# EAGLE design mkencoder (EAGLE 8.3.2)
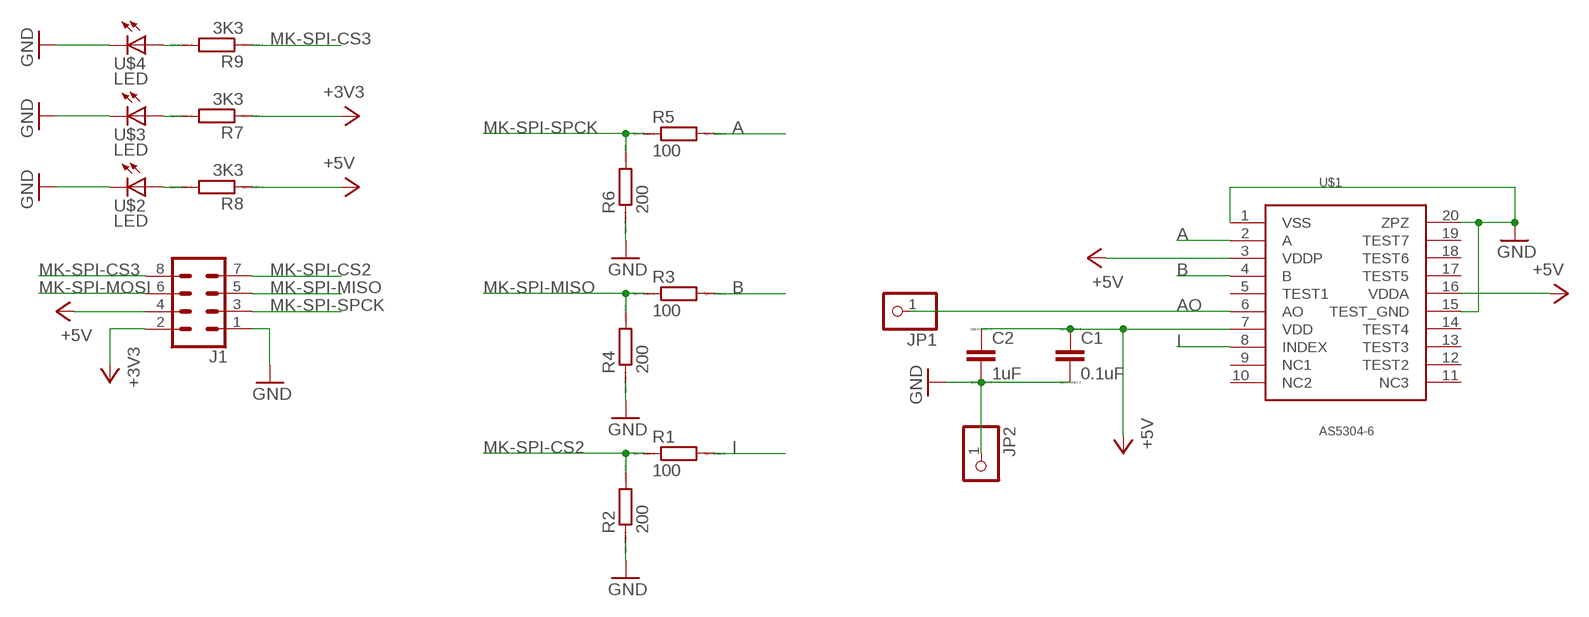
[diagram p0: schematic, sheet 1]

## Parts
C1  0.1uF  C  [C0805]
C2  1uF  C  [C0805]
J1  CONN_04X2SHROUDED-SQUISH  [2X4-SHROUDED-SQUISH]
JP1  PINHD-1X1  [1X01]
JP2  PINHD-1X1  [1X01]
R1  100  RR1206  [R1206]
R2  200  RR1206  [R1206]
R3  100  RR1206  [R1206]
R4  200  RR1206  [R1206]
R5  100  RR1206  [R1206]
R6  200  RR1206  [R1206]
R7  3K3  RR1206  [R1206]
R8  3K3  RR1206  [R1206]
R9  3K3  RR1206  [R1206]
U$1  AS5304-6  [TSSOP20-08THIN]
U$2  LED  [LED1206]
U$3  LED  [LED1206]
U$4  LED  [LED1206]

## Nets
+3V3: J1.2 R7.1
+5V: C1.1 C2.1 J1.4 R8.1 U$1.3(VDDP) U$1.7(VDD) U$1.16(VDDA)
A: R5.2 U$1.2(A)
AO: JP1.1 U$1.6(AO)
B: R3.2 U$1.4(B)
GND: C1.2 C2.2 J1.1 JP2.1 R2.1 R4.1 R6.1 U$1.1(VSS) U$1.15(TEST_GND) U$1.20(ZPZ) U$2.2(C) U$3.2(C) U$4.2(C)
I: R1.2 U$1.8(INDEX)
MK-SPI-CS2: J1.7 R1.1 R2.2
MK-SPI-CS3: J1.8 R9.1
MK-SPI-MISO: J1.5 R3.1 R4.2
MK-SPI-MOSI: J1.6
MK-SPI-SPCK: J1.3 R5.1 R6.2
N$1: R8.2 U$2.1(A)
N$2: R7.2 U$3.1(A)
N$5: R9.2 U$4.1(A)
Unconnected: U$1.5(TEST1) U$1.9(NC1) U$1.10(NC2) U$1.11(NC3) U$1.12(TEST2) U$1.13(TEST3) U$1.14(TEST4) U$1.17(TEST5) U$1.18(TEST6) U$1.19(TEST7)

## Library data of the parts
C1 C2 = eagle-ltspice:C: CAPACITOR, European symbol; SPICEMODEL: NONE; SPICEPREFIX: C
J1 = fab:CONN_04X2: Multi connection point. Often used as Generic Header-pin footprint for 0.1 inch spaced/style header connections On any of the 0.1 inch spaced packages, you can populate with these: Break Away Headers - Straight (PRT-00116) Break Away Male Headers - Right Angle (PRT-00553) Female Headers (PRT-00115)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
JP1 JP2 = pinhead:PINHD-1X1: PIN HEADER
R1-R9 = eagle-ltspice:R: RESISTOR, European symbol; SPICEMODEL: NONE; SPICEPREFIX: R
U$1 = fab:AS5304-6
U$2-U$4 = fab:LED: LED

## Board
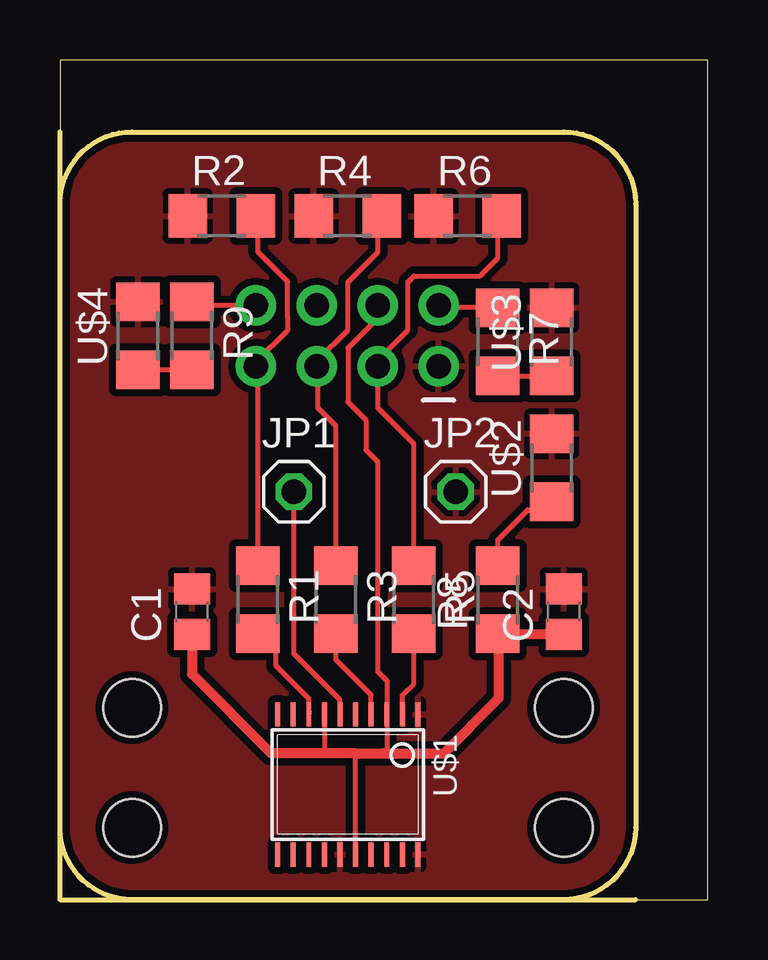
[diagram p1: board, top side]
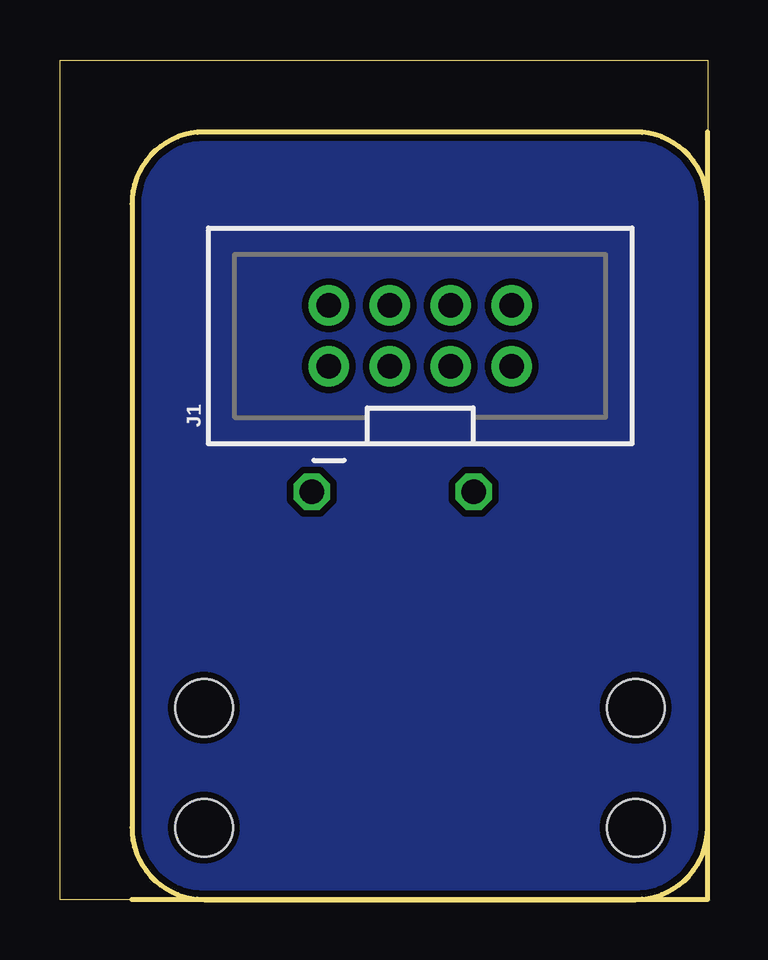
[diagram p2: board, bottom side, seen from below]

Size 27 x 35 mm. Coordinates in mm from the lower left corner, seen from the top.
Outline: 0,3 0,0 3,0
Outline: 0,3 0,29
Outline: 0,29 0,32 0,35 27,35 27,0 24,0 21,0
Outline: 3,0 21,0
Outline: 0,29 arc-90 3,32 21,32 arc-90 24,29 24,3 arc-90 21,0
Outline: 3,0 arc-90 0,3
Copper layers (1*16): Top 0.035mm / dielectric 1.5mm / Bottom 0.035mm
Design rules "default *": minimum track width 7mil, minimum drill 0.35mm, track to track 11mil, track to pad 11mil, pad to pad 11mil, via to via 11mil, smd to smd 11mil, copper to edge 11mil, drill to drill 11mil, minimum pad ring 10mil, minimum via ring 8mil, stop-mask expansion 4mil, vias tented up to drill 0mil, thermal gap 10mil
Holes 2.4 mm at 3,3 21,3 3,8 21,8
Milling: 8 lines

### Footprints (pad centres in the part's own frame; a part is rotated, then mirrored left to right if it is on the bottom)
C0805 = smd 1.3 x 1.5: 1 -0.95,0; 2 0.95,0
2X4-SHROUDED-SQUISH = drill 1.016 pad 1.676: 1 -1.27,2.54; 2 1.27,2.54; 3 -1.27,0; 4 1.27,0; 5 -1.27,-2.54; 6 1.27,-2.54; 7 -1.27,-5.08; 8 1.27,-5.08
1X01 = drill 1.016 octagon: 1 0,0
R1206 = smd 1.6 x 1.803: 1 -1.422,0; 2 1.422,0
TSSOP20-08THIN = smd 0.203 x 1.016: 1 -2.925,-2.918; 2 -2.275,-2.918; 3 -1.625,-2.918; 4 -0.975,-2.918; 5 -0.325,-2.918; 6 0.325,-2.918; 7 0.975,-2.918; 8 1.625,-2.918; 9 2.275,-2.918; 10 2.925,-2.918; 11 2.925,2.918; 12 2.275,2.918; 13 1.625,2.918; 14 0.975,2.918; 15 0.325,2.918; 16 -0.325,2.918; 17 -0.975,2.918; 18 -1.625,2.918; 19 -2.275,2.918; 20 -2.925,2.918
LED1206 = smd 1.6 x 1.803: 1 -1.422,0; 2 1.422,0

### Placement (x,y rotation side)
C1  5.5,12 90 top
C2  21,12 90 top
J1  13.25,23.5 90 bottom
JP1  9.75,17 0 top
JP2  16.5,17 0 top
R1  8.25,12.5 270 top
R2  6.75,28.5 0 top
R3  11.5,12.5 270 top
R4  12,28.5 0 top
R5  14.75,12.5 270 top
R6  17,28.5 0 top
R7  18.25,23.25 270 top
R8  18.25,12.5 90 top
R9  5.5,23.5 270 top
U$1  12,4.8 180 top
U$2  20.5,18 90 top
U$3  20.5,23.25 90 top
U$4  3.25,23.5 90 top

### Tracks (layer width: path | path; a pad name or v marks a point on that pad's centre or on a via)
+3V3
  Top 0.2: R7.1 15.89,24.67 J1.2
+5V
  Top 0.2: J1.4 13.25,24.25 12,23 12,20.75 12.75,20 12.75,18.75 13.25,18.25 13.25,9.5 13.62,9.12 U$1.3 13.62,6.22 13.5,6.1 | U$1.7 11.03,6.12 11,6.1 | U$1.16 12.32,6.08 12.3,6.1
  Top 0.406: C1.1 5.5,9.4 8.8,6.1 11,6.1 12.3,6.1 13.5,6.1 16,6.1 18.3,8.4 18.3,11.03 R8.1 20.97,11.08 C2.1
A
  Top 0.2: U$1.2 14.28,8.53 14.75,9 R5.2
AO
  Top 0.2: 11.68,7.83 U$1.6 11.68,8.32 9.75,10.25 JP1.1
B
  Top 0.2: U$1.4 12.97,8.53 11.5,10 R3.2
GND
  pour Top (isolate 0.305): 0,32 0,0 24,0 24,32
I
  Top 0.2: 10.38,7.88 U$1.8 10.38,8.38 9,9.75 9,10.33 R1.2
MK-SPI-CS2
  Top 0.2: R1.1 8.25,22.15 J1.7 8.17,22.42 9.5,23.75 9.5,24.26 9.49,24.27 9.49,25.76 8.25,27 8.25,28.42 R2.2
MK-SPI-CS3
  Top 0.2: J1.8 5.65,24.77 R9.1
MK-SPI-MISO
  Top 0.2: R3.1 11.5,19.75 10.75,20.5 10.75,22.19 J1.5 10.71,22.46 12,23.75 12,25.75 13.25,27 13.25,28.33 R4.2
MK-SPI-SPCK
  Top 0.2: R6.2 18.25,28.33 18.25,26.75 17.5,26 14.75,26 14.5,25.75 14.5,23.75 13.25,22.5 J1.3 13.25,20.5 14.75,19 R5.1
N$1
  Top 0.2: R8.2 18.25,15 18.75,15.5 19.5,16.25 20.17,16.25 U$2.1
N$2
  Top 0.2: R7.2 U$3.1
N$3
  pour Bottom (isolate 0.01): 2.75,0 2,0 1.75,0.25 1.5,0.25 0.75,1 0.25,1.5 0.25,1.75 0,2 0,29.25 0,30 0.25,30.25 0.25,30.5 0.75,31 1.5,31.75 1.75,31.75 2,32 21.25,32 22,32 22.25,31.75 22.5,31.75 23.75,30.5 23.75,30.25 24,30 24,2.75 24,2 23.75,1.75 23.75,1.25 23,0.5 22.75,0.5 22.5,0.25 22.25,0.25 22,0
N$5
  Top 0.2: R9.2 U$4.1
